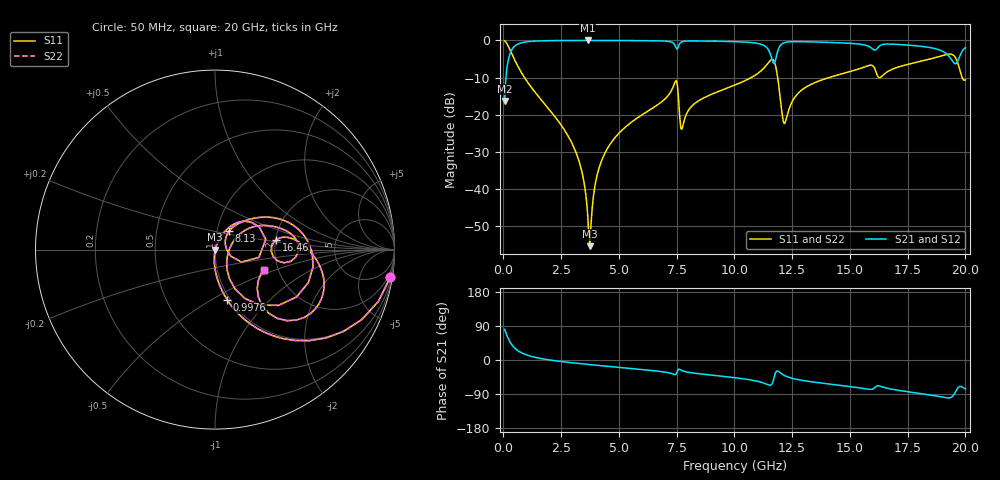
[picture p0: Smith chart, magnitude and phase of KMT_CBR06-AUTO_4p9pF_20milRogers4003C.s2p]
! Data measured by Modelithics Inc. support@modelithics.com 813-866-6335
! KEMET CBR06-AUTO 4.9pF, Pad Width= 0.851mm, Pad Length= 0.64mm, Pad Gap= 0.62mm, 20mil Rogers 4003C substrate Data, January 2022
# hz S ma R 50
! 2 Port Network Data from SP1.SP block
! freq  magS11  angS11  magS21  angS21  magS12  angS12  magS22  angS22
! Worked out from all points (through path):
!   401 points, 50 MHz to 20 GHz, reference 50 ohm
!   highest |S21| = -0.02 dB at 3.641 GHz (marker M1); lowest = -16.3 dB at 50 MHz (marker M2)
!   group delay of S21, straight-line fit = 15.4 ps
!   lowest |S11| = -55.4 dB at 3.741 GHz (marker M3), VSWR 1.00, Z = 50.2 + j0.00501 ohm
!   |S11| at or under -10 dB: 910.9 MHz to 10.73 GHz (9.818 GHz wide, 169 % of centre); 11.87 GHz to 14.1 GHz (2.227 GHz wide, 17.2 % of centre); 19.86 GHz to end of sweep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
!   |S22| runs from -55.4 to -0.1 dB; largest |S21 - S12| = 0
!   S11 on the Smith chart (normalised r, x): 50 MHz: 1, -13; 997.6 MHz: 0.97, -0.59; 8.13 GHz: 1.14, +0.24; 16.46 GHz: 2.02, +0.25; 20 GHz: 1.69, -0.41
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5e7  0.9881 -9.0  0.1533 81.0  0.1533 81.0  0.9881 -9.0
3.4925e8  0.6747 -48.6  0.7374 41.3  0.7374 41.3  0.6747 -48.6
9.97625e8  0.2879 -76.3  0.9567 13.5  0.9567 13.5  0.2879 -76.3
2.74325e9  0.05528 -94.3  0.9969 -5.8  0.9969 -5.8  0.05528 -94.3
3.391625e9  0.01728 -94.8  0.9982 -10.0  0.9982 -10.0  0.01728 -94.8
3.641e9  0.004765 -81.6  0.9982 -11.6  0.9982 -11.6  0.004765 -81.6
3.74075e9  0.001697 1.7  0.9982 -12.2  0.9982 -12.2  0.001697 1.7
4.04e9  0.0146 69.3  0.998 -14.0  0.998 -14.0  0.0146 69.3
4.488875e9  0.03452 70.4  0.9974 -16.6  0.9974 -16.6  0.03452 70.4
6.73325e9  0.14 58.4  0.9855 -29.8  0.9855 -29.8  0.14 58.4
7.4315e9  0.2767 27.7  0.8561 -38.7  0.8561 -38.7  0.2767 27.7
7.73075e9  0.06395 25.0  0.9598 -27.9  0.9598 -27.9  0.06395 25.0
8.12975e9  0.128 52.7  0.9833 -33.6  0.9833 -33.6  0.128 52.7
1.0025e10  0.2511 41.8  0.9614 -46.8  0.9614 -46.8  0.2511 41.8
1.127188e10  0.423 22.2  0.8565 -61.0  0.8565 -61.0  0.423 22.2
1.167088e10  0.5519 -19.4  0.5042 -57.1  0.5042 -57.1  0.5519 -19.4
1.216962e10  0.07572 -11.3  0.9331 -41.1  0.9331 -41.1  0.07572 -11.3
1.336662e10  0.2604 30.0  0.9545 -57.7  0.9545 -57.7  0.2604 30.0
1.645888e10  0.3458 9.1  0.8859 -72.1  0.8859 -72.1  0.3458 9.1
1.670825e10  0.3922 10.2  0.8926 -75.9  0.8926 -75.9  0.3922 10.2
1.935162e10  0.6534 -27.4  0.5786 -99.2  0.5786 -99.2  0.6534 -27.4
2e10  0.2949 -22.1  0.7989 -76.6  0.7989 -76.6  0.2949 -22.1
